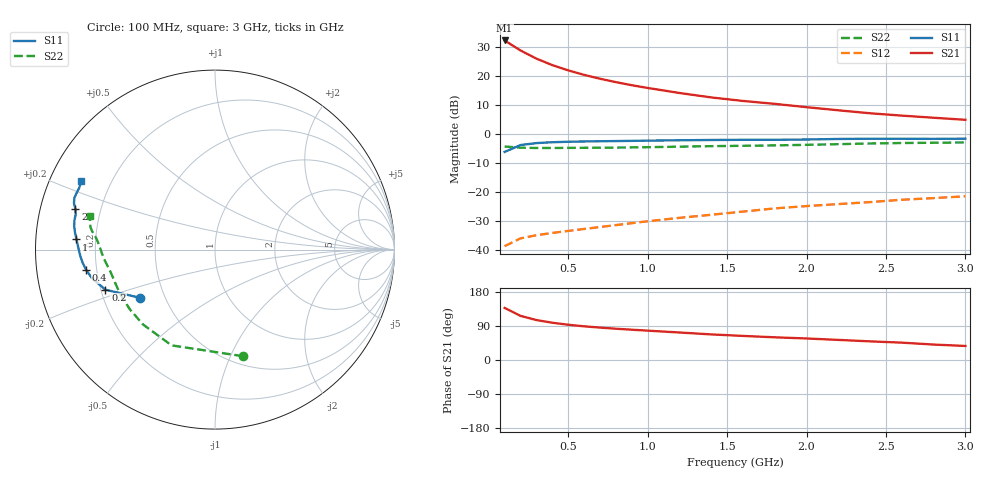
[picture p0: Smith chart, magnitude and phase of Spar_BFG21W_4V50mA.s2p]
! Filename: 450bfg21.001
! Title: BFG21W
! Bias: Vce=4V; Ic=50mA
! Company: NXP Semiconductors NL
! User: Quality&Reliability T&D
! Measure time: 10 Nov 1999 / 11:45:17
#  MHz  S  MA  R 50
! Freq  S11  S21  S12  S22  :
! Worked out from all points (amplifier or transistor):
!   20 points, 100 MHz to 3 GHz, reference 50 ohm
!   highest |S21| = 32.3 dB at 100 MHz (marker M1)
!   |S21| within 3 dB of that: start of sweep to 187.2 MHz
!   unconditionally stable (mu >= 1): 849.2 MHz to end of sweep
!   at 400 MHz: K = 0.71, MSG = 28.9 dB, |S12| = -34.0 dB
!   at 1.2 GHz: K = 1.07, MAG = 19.9 dB, |S12| = -28.8 dB
!   at 3 GHz: K = 1.05, MAG = 11.8 dB, |S12| = -21.4 dB
!   S11 on the Smith chart (normalised r, x): 100 MHz: 0.36, -0.26; 200 MHz: 0.22, -0.17; 400 MHz: 0.16, -0.08; 1 GHz: 0.13, +0.04; 2 GHz: 0.11, +0.14; 3 GHz: 0.09, +0.24
100  0.4954 -147.1  41.06 137.5  0.01182 45.9  0.6141 -75.3
200  0.6501 -159.9  27.63 116.5  0.0161 40.2  0.5858 -114.4
300  0.703 -166.8  19.98 105.5  0.01825 40.5  0.5787 -133.8
400  0.727 -171.1  15.46 98.3  0.01997 42.6  0.5794 -144.8
500  0.7409 -174.3  12.55 93.1  0.02163 45.4  0.5813 -151.9
600  0.7497 -176.8  10.5 88.9  0.02337 48.3  0.5835 -156.9
700  0.7561 -178.9  9.019 85.5  0.02524 51.4  0.5855 -160.6
800  0.7616 179.2  7.871 82.5  0.02722 54.1  0.5882 -163.7
900  0.7675 177.4  6.971 80.0  0.02937 56.9  0.5923 -166.4
1000  0.7741 175.8  6.254 77.4  0.03172 58.8  0.5974 -168.8
1200  0.7863 172.9  5.124 72.6  0.03634 62.1  0.6103 -172.6
1400  0.795 170.6  4.295 67.5  0.04101 64.2  0.6224 -175.7
1600  0.8 168.3  3.735 63.6  0.04659 66.1  0.6311 -178.3
1800  0.8005 165.8  3.327 59.9  0.05282 67.5  0.6414 178.9
2000  0.8099 163.8  2.918 56.8  0.05788 68.9  0.6557 175.9
2200  0.8276 161.7  2.578 53.0  0.06268 69.5  0.6734 173.4
2400  0.8349 159.8  2.292 49.2  0.06779 69.3  0.6919 171.5
2600  0.8334 157.9  2.088 45.8  0.07441 68.9  0.705 169.8
2800  0.8312 155.5  1.919 40.7  0.07942 67.6  0.7121 167.7
3000  0.8364 153.0  1.769 37.1  0.08533 67.0  0.7216 165.1
